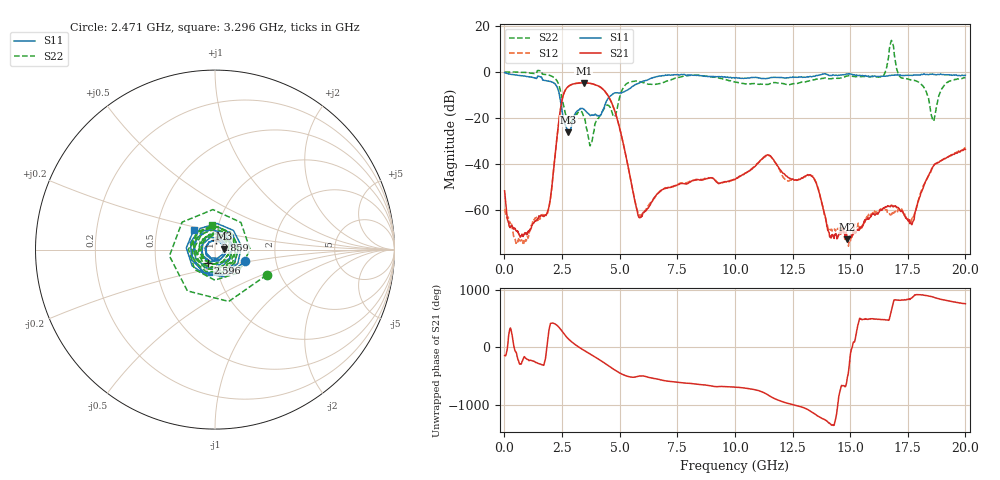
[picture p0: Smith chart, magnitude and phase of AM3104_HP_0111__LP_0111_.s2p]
!Created with skrf (http://scikit-rf.org).
# Hz S RI R 50.0
!freq ReS11 ImS11 ReS21 ImS21 ReS12 ImS12 ReS22 ImS22
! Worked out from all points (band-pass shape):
!   1601 points, 10 MHz to 20 GHz, reference 50 ohm
!   highest |S21| = -4.77 dB at 3.446 GHz (marker M1); lowest = -72.6 dB at 14.88 GHz (marker M2)
!   |S21| within 3 dB of the highest: 2.652 GHz to 4.303 GHz (1.65 GHz wide, 47.5 % of centre)
!   lowest |S11| = -26.2 dB at 2.771 GHz (marker M3), VSWR 1.10, Z = 55.1 + j0.592 ohm
!   |S11| at or under -10 dB: 2.388 GHz to 4.654 GHz (2.267 GHz wide, 64.4 % of centre)
!   |S22| runs from -32.1 to 13.6 dB; largest |S21 - S12| = 0.036
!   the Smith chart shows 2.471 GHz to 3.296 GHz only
!   S11 on the Smith chart (normalised r, x): 2.471 GHz: 1.39, -0.19; 2.596 GHz: 0.92, -0.13; 2.859 GHz: 1.00, +0.11; 3.296 GHz: 0.77, +0.17
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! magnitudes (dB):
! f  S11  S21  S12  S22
! 10 MHz  -0.3  -51.6  -59.7  -0.1
! 722.1 MHz  -1.7  -71.3  -73.2  -0.3
! 1.809 GHz  -3.8  -62.3  -62.0  -1.2
! 2.471 GHz  -14.9  -13.9  -13.9  -9.9
! 2.596 GHz  -21.7  -8.9  -8.9  -16.0
! 2.771 GHz  -26.2  -6.4  -6.4  -21.8
! 2.859 GHz  -25.5  -5.8  -5.8  -22.1
! 3.296 GHz  -15.9  -4.8  -4.9  -17.2
! 3.346 GHz  -15.9  -4.8  -4.9  -17.3
! 3.446 GHz  -16.2  -4.8  -4.8  -19.6
! 3.733 GHz  -19.0  -5.0  -5.0  -31.7
! 4.683 GHz  -9.8  -14.1  -14.2  -18.0
! 5.845 GHz  -4.9  -63.2  -62.2  -4.2
! 6.682 GHz  -1.9  -52.6  -52.5  -5.3
! 10.01 GHz  -2.7  -46.8  -46.6  -4.4
! 13.34 GHz  -2.1  -45.3  -45.2  -3.7
! 14.1 GHz  -1.6  -71.1  -68.0  -3.0
! 14.88 GHz  -0.9  -72.6  -72.8  -1.9
! 16.68 GHz  -1.6  -58.4  -61.3  7.2
! 17.68 GHz  -1.6  -66.3  -63.9  -3.7
! 18.6 GHz  -1.1  -41.1  -41.4  -21.3
! 20 GHz  -1.5  -33.6  -33.0  -2.5
